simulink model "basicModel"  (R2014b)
settings: Solver=ode45  StartTime=0.0  StopTime=1000  RelTol=1e-3

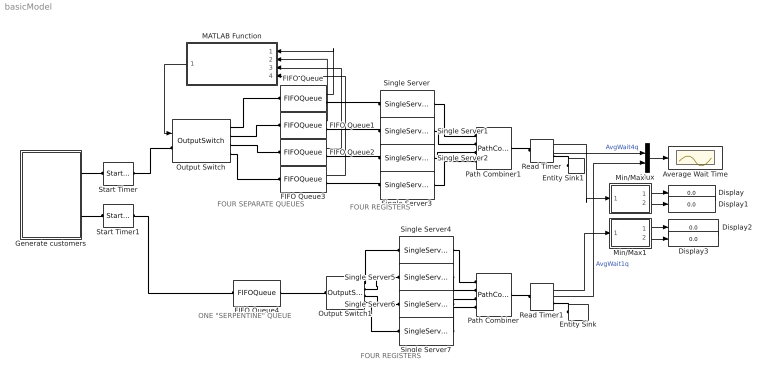
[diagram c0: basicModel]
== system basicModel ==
  note: FOUR SEPARATE QUEUES
  note: ONE "SERPENTINE" QUEUE
  note: FOUR REGISTERS
  note: FOUR REGISTERS
  Average Wait Time : Scope
  Display{,1..3} (4 alike) : Display
  Entity Sink : EntitySink
  Entity Sink1 : EntitySink
  FIFO Queue{,1..3} (4 alike) : FIFOQueue  Capacity=inf  StatNumberInBlock=on
  FIFO Queue4 : FIFOQueue  Capacity=inf
  Generate customers : Subsystem
  MATLAB Function : MATLAB Function  TreatAsAtomicUnit=on
  Min/Max : Subsystem  TreatAsAtomicUnit=on
  Min/Max1 : Subsystem  TreatAsAtomicUnit=on
  Mux : Mux  Inputs=2
  Output Switch : OutputSwitch  NumberOutputPorts=4  SwitchingCriterion=From signal port p  InitialConditionsOpt=on
  Output Switch1 : OutputSwitch  NumberOutputPorts=4
  Path Combiner : PathCombiner  NumberInputPorts=4
  Path Combiner1 : PathCombiner  NumberInputPorts=4
  Read Timer : ReadTimer  StatTimeElapsed=on  StatAverageTimeElapsed=on
  Read Timer1 : ReadTimer  TimerTag=T2  StatTimeElapsed=on  StatAverageTimeElapsed=on
  Single Server{,1..7} (8 alike) : SingleServer  ServiceTimeFrom=Attribute  AttributeName=sTime
  Start Timer : StartTimer
  Start Timer1 : StartTimer  TimerTag=T2
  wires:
  FIFO Queue/1 -> MATLAB Function/1(n1)
  FIFO Queue1/1 -> MATLAB Function/2(n2)
  FIFO Queue2/1 -> MATLAB Function/3(n3)
  FIFO Queue3/1 -> MATLAB Function/4(n4)
  MATLAB Function/1(sq) -> Output Switch/1
  Mux/1 -> Average Wait Time/1
  Read Timer/2 -> Mux/1  "AvgWait4q"
  Read Timer1/2 -> Mux/2  "AvgWait1q"
  Read Timer/1 -> Min/Max/1(u)
  Read Timer1/1 -> Min/Max1/1(u)
  Min/Max/1(min) -> Display/1
  Min/Max/2(max) -> Display1/1
  Min/Max1/1(min) -> Display2/1
  Min/Max1/2(max) -> Display3/1
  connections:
  Output Switch/RConn1 -- FIFO Queue/LConn1
  Output Switch/RConn2 -- FIFO Queue1/LConn1
  Output Switch/RConn3 -- FIFO Queue2/LConn1
  Output Switch/RConn4 -- FIFO Queue3/LConn1
  Start Timer1/RConn1 -- FIFO Queue4/LConn1
  Single Server/LConn1 -- FIFO Queue/RConn1
  Single Server1/LConn1 -- FIFO Queue1/RConn1
  Single Server2/LConn1 -- FIFO Queue2/RConn1
  Single Server3/LConn1 -- FIFO Queue3/RConn1
  Output Switch1/RConn1 -- Single Server4/LConn1
  Output Switch1/RConn2 -- Single Server5/LConn1
  Output Switch1/RConn3 -- Single Server6/LConn1
  Output Switch1/RConn4 -- Single Server7/LConn1
  FIFO Queue4/RConn1 -- Output Switch1/LConn1
  Single Server4/RConn1 -- Path Combiner/LConn1
  Single Server5/RConn1 -- Path Combiner/LConn2
  Single Server6/RConn1 -- Path Combiner/LConn3
  Single Server7/RConn1 -- Path Combiner/LConn4
  Entity Sink/LConn1 -- Read Timer1/RConn1
  Entity Sink1/LConn1 -- Read Timer/RConn1
  Single Server/RConn1 -- Path Combiner1/LConn1
  Single Server1/RConn1 -- Path Combiner1/LConn2
  Single Server2/RConn1 -- Path Combiner1/LConn3
  Single Server3/RConn1 -- Path Combiner1/LConn4
  Start Timer/RConn1 -- Output Switch/LConn1
  Read Timer/LConn1 -- Path Combiner1/RConn1
  Read Timer1/LConn1 -- Path Combiner/RConn1
  Generate customers/RConn1 -- Start Timer/LConn1
  Generate customers/RConn2 -- Start Timer1/LConn1

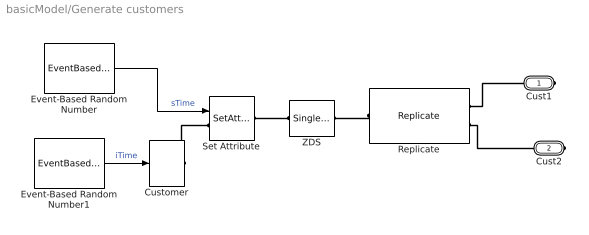
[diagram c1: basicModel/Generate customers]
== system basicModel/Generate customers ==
  Customer : TimeBasedEntityGenerator  GenerateEntitiesUpon=Intergeneration time from port t  Distribution=Exponential  InitialSeed=35250  Mean=0.9  GenerateEntityAtSimulationStart=off
  Event-Based Random Number : EventBasedRandomNumber  meanExp=2  Seed=32033
  Event-Based Random Number1 : EventBasedRandomNumber  Seed=35250
  Replicate : Replicate  NumberOutputPorts=2
  Set Attribute : SetAttribute  AttributeName=sTime  AttributeFrom=Signal port  EvaluatedAttributeValue={ []}
  ZDS : SingleServer  ServiceTime=0  AttributeName=sTime
  Cust1 : PMIOPort  Port=1  Side=Right
  Cust2 : PMIOPort  Port=2  Side=Right
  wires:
  Event-Based Random Number/1 -> Set Attribute/1  "sTime"
  Event-Based Random Number1/1 -> Customer/1  "iTime"
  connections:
  Replicate/LConn1 -- ZDS/RConn1
  Replicate/RConn1 -- Cust1/RConn1
  Customer/RConn1 -- Set Attribute/LConn1
  Set Attribute/RConn1 -- ZDS/LConn1
  Replicate/RConn2 -- Cust2/RConn1

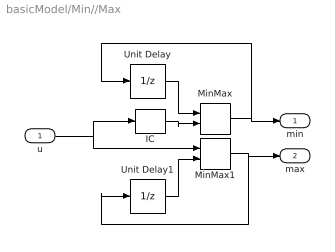
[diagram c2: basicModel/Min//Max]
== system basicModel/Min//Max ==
  u : Inport
  IC : InitialCondition  Value=100
  MinMax : MinMax  Inputs=2
  MinMax1 : MinMax  Function=max  Inputs=2
  Unit Delay : UnitDelay  InitialCondition=100  SampleTime=-1
  Unit Delay1 : UnitDelay  SampleTime=-1
  min : Outport
  max : Outport  Port=2
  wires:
  Unit Delay1/1 -> MinMax1/2
  MinMax1/1 -> Unit Delay1/1, max/1
  Unit Delay/1 -> MinMax/1
  MinMax/1 -> Unit Delay/1, min/1
  u/1 -> MinMax1/1, IC/1
  IC/1 -> MinMax/2

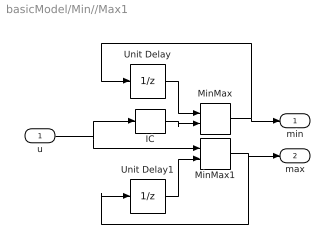
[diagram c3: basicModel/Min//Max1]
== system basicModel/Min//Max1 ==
  u : Inport
  IC : InitialCondition  Value=100
  MinMax : MinMax  Inputs=2
  MinMax1 : MinMax  Function=max  Inputs=2
  Unit Delay : UnitDelay  InitialCondition=100  SampleTime=-1
  Unit Delay1 : UnitDelay  SampleTime=-1
  min : Outport
  max : Outport  Port=2
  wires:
  IC/1 -> MinMax/2
  u/1 -> IC/1, MinMax1/1
  MinMax/1 -> min/1, Unit Delay/1
  Unit Delay/1 -> MinMax/1
  MinMax1/1 -> max/1, Unit Delay1/1
  Unit Delay1/1 -> MinMax1/2

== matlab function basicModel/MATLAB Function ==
function sq = shortestQueue(n1,n2,n3,n4)
%#codegen

[~,sq] = min([n1, n2, n3, n4]);
